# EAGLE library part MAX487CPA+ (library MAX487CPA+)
MAX487CPA+, Line Transceiver, RS-485, RS-422 Differential, 5 V, 8-Pin PDIP Source: Datasheet
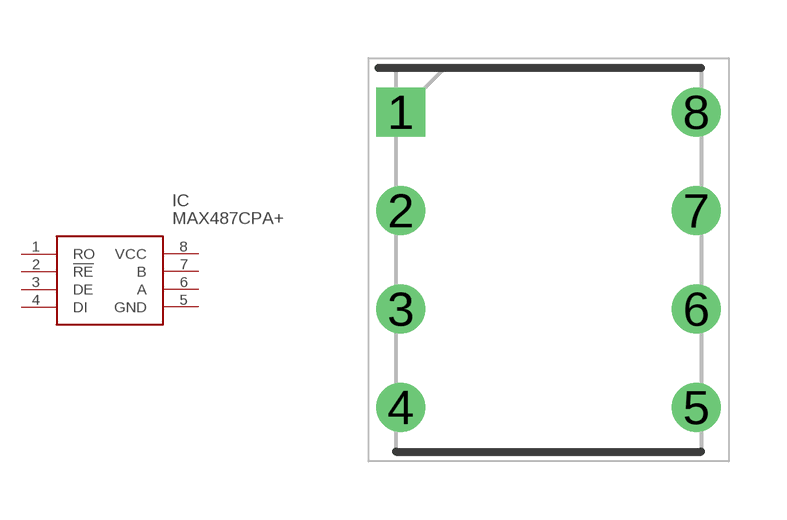
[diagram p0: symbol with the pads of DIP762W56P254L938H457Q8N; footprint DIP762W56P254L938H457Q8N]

Designator prefix IC

## MAX487CPA+ (Arrow_Part_Number: MAX487CPA+; Arrow_Price-Stock: https://www.arrow.com/en/products/max487cpa/maxim-integrated?region=nac; Description: MAX487CPA+, Line Transceiver, RS-485, RS-422 Differential, 5 V, 8-Pin PDIP; Height: 4.572mm; Manufacturer_Name: Maxim Integrated; Manufacturer_Part_Number: MAX487CPA+; Mouser_Part_Number: 700-MAX487CPA; Mouser_Price-Stock: https://www.mouser.co.uk/ProductDetail/Maxim-Integrated/MAX487CPA%2b?qs=1THa7WoU59FIe2IfA72xDw%3D%3D)  [DIP762W56P254L938H457Q8N]
1  RO
2  !RE
3  DE
4  DI
5  GND
6  A
7  B
8  VCC

## Footprint DIP762W56P254L938H457Q8N (pad centres in mm)
MAX487CPA+
drill 0.76 pad 1.16 square: 1 -3.81,3.81
drill 0.76 pad 1.16: 2 -3.81,1.27; 3 -3.81,-1.27; 4 -3.81,-3.81; 5 3.81,-3.81; 6 3.81,-1.27; 7 3.81,1.27; 8 3.81,3.81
